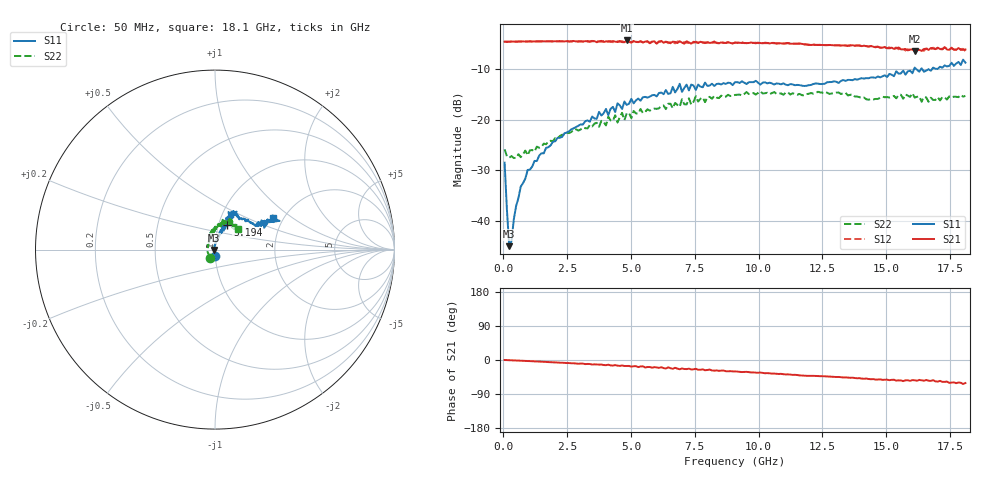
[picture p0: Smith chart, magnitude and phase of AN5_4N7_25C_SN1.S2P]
! Network Analyzer HP8720D.06.14 Serial No. US36140669
!  5 Jul 2005  06:43:14
! Frequency  S11  S21  S12  S22
# HZ  S  DB R 50
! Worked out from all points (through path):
!   201 points, 50 MHz to 18.1 GHz, reference 50 ohm
!   highest |S21| = -4.29 dB at 4.833 GHz (marker M1); lowest = -6.4 dB at 16.11 GHz (marker M2)
!   group delay of S21, straight-line fit = 9.56 ps
!   lowest |S11| = -45.0 dB at 230.5 MHz (marker M3), VSWR 1.01, Z = 49.5 - j0.256 ohm
!   |S11| at or under -10 dB: start of sweep to 16.09 GHz; 16.18 GHz to 16.36 GHz (175.1 MHz wide, 1.08 % of centre); 16.41 GHz to 16.65 GHz (238.6 MHz wide, 1.44 % of centre)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
!   |S22| runs from -27.6 to -14.4 dB; largest |S21 - S12| = 0.029
!   S11 on the Smith chart (normalised r, x): 50 MHz: 0.99, -0.07; 5.194 GHz: 1.10, +0.31; 18.1 GHz: 1.76, +0.72
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5e7  -28.49 -93.3  -4.54 0.0  -4.52 0.3  -25.85 -119.6
2.305e8  -45.02 -152.5  -4.54 -0.4  -4.55 -0.2  -27.51 -176.6
3.2075e8  -43.95 141.9  -4.50 -0.6  -4.52 -0.6  -27.19 175.1
4.11e8  -39.67 113.9  -4.53 -1.1  -4.50 -0.9  -27.57 170.4
6.8175e8  -33.23 95.6  -4.49 -1.9  -4.50 -1.6  -27.41 155.2
9.525e8  -29.93 87.9  -4.48 -2.7  -4.48 -2.5  -27.01 144.3
2.12575e9  -23.56 75.8  -4.47 -6.8  -4.46 -6.6  -23.70 116.1
3.1185e9  -20.93 73.3  -4.50 -9.6  -4.52 -10.0  -21.53 109.8
4.021e9  -17.85 71.0  -4.47 -13.7  -4.54 -12.4  -21.11 100.6
4.382e9  -18.47 68.8  -4.53 -13.3  -4.50 -14.7  -19.09 99.5
4.47225e9  -16.74 64.9  -4.61 -14.9  -4.46 -13.7  -20.54 102.1
4.83325e9  -17.05 72.8  -4.29 -15.8  -4.49 -16.5  -18.70 88.8
5.19425e9  -16.17 63.8  -4.60 -16.3  -4.47 -16.3  -18.73 96.3
6.09675e9  -14.69 65.4  -4.56 -20.7  -4.46 -20.1  -17.73 83.3
6.7285e9  -14.58 70.2  -4.59 -20.5  -4.86 -21.5  -16.66 75.2
6.909e9  -12.87 66.8  -4.45 -24.4  -4.59 -22.4  -17.43 74.1
6.99925e9  -14.47 66.8  -4.73 -22.3  -4.86 -24.3  -15.91 74.7
9.075e9  -12.55 62.7  -4.73 -30.1  -4.71 -30.0  -15.07 63.5
1.21435e10  -12.91 50.4  -5.14 -41.8  -5.10 -41.6  -14.81 65.5
1.512175e10  -10.92 28.6  -5.85 -53.3  -5.65 -52.4  -15.59 57.7
1.61145e10  -9.67 26.8  -6.40 -53.6  -6.02 -53.6  -15.59 50.0
1.81e10  -8.69 28.9  -6.08 -60.8  -6.37 -61.3  -15.27 42.0
